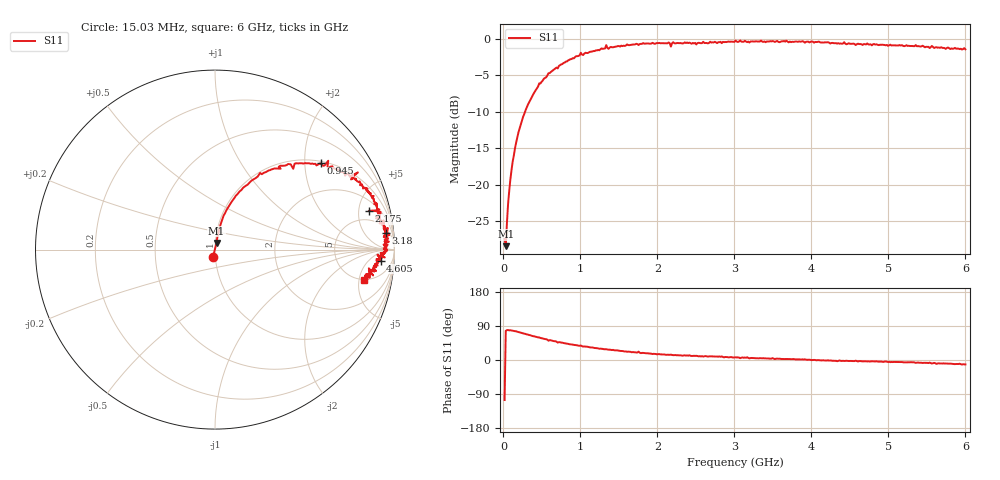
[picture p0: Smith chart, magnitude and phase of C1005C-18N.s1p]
!	Network	Analyzer	HP8753E.07.74:	Oct	30	2002	Serial	No.	JP38451487
!	Hewlett-Packard
!	7	Sep	2009	8:51:12
!	Frequency	S11
#	HZ	S	RI	R	50
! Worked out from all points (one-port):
!   400 points, 15.03 MHz to 6 GHz, reference 50 ohm
!   lowest |S11| = -28.4 dB at 30.03 MHz (marker M1), VSWR 1.08, Z = 50.7 + j3.77 ohm
!   |S11| at or under -10 dB: start of sweep to 280.1 MHz
!   S11 on the Smith chart (normalised r, x): 15.03 MHz: 0.97, -0.08; 945 MHz: 1.05, +2.40; 2.175 GHz: 3.26, +6.44; 3.18 GHz: 8, +17; 4.605 GHz: 15, -13; 6 GHz: 4.85, -5.85
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1.502992e7  -0.0115 -0.0411
3.002985e7  0.00869 0.0371
6.00297e7  0.014 0.0727
1.050295e8  0.0266 0.124
1.650292e8  0.0478 0.189
2.400288e8  0.0891 0.261
4.650277e8  0.251 0.427
7.650262e8  0.468 0.481
9.450253e8  0.588 0.481
1.320023e9  0.755 0.409
1.335023e9  0.796 0.43
1.365023e9  0.758 0.391
1.515022e9  0.808 0.359
1.725021e9  0.869 0.313
1.755021e9  0.839 0.342
1.785021e9  0.877 0.287
1.93502e9  0.902 0.255
2.145019e9  0.916 0.224
2.175019e9  0.857 0.216
2.205019e9  0.923 0.209
2.265019e9  0.913 0.205
3.015015e9  0.964 0.119
3.180014e9  0.952 0.0916
3.765011e9  0.95 0.0413
4.515007e9  0.922 -0.0398
4.605007e9  0.923 -0.0618
5.265004e9  0.89 -0.0951
6e9  0.829 -0.171
